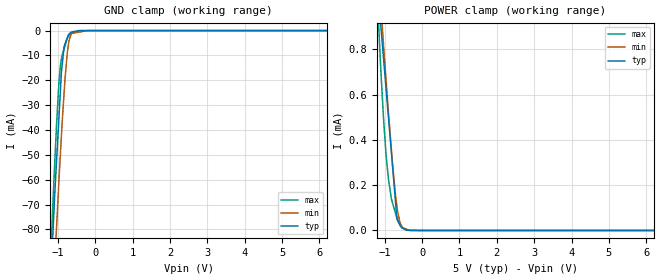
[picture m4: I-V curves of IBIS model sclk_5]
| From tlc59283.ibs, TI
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|   sclk_5 Model
[Model]   sclk_5
Model_type   Input
Vinl = 1.5
Vinh = 3.5
|   typ   min   max
C_comp   5.295e-13   5.058e-13   5.549e-13
| Where nom  PVT is Nominal Process, 5V, 27C
|   Fast PVT is Strong Process,  5.5V, -40C
|   Slow PVT is Weak Process,   4.5V, 125C
[Voltage Range]   5   4.5   5.5
|Ambient Temperature   25   85   -40
|Junction Temperature
[Temperature Range]   27   125   -40
[Power Clamp Reference]   5   4.5   5.5
[GND Clamp Reference]   0   0   0
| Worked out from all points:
|   GND clamp passes 1 mA (typ) near -0.67 V on its own axis
|   POWER clamp passes 1 mA (typ) near -1.15 V on its own axis
[GND Clamp]
|   Voltage   I(typ)   I(min)   I(max)
-5V       -1.598A    -1.521A    -1.69A
-1.373V   -164.7mA   -186.9mA   -158.6mA
-1.14V    -84.95mA   -112.5mA   -73.36mA
-1.122V   -79.17mA   -106.7mA   -66.76mA
-1.034V   -53.01mA   -79.68mA   -38.29mA
-973.5mV  -36.35mA   -61.85mA   -22.17mA
-929.5mV  -24.23mA   -49.72mA   -14.25mA
-900mV    -16.47mA   -41.67mA   -11.16mA
-830mV    -6.402mA   -24.98mA   -7.326mA
-742.5mV  -2.72mA    -8.782mA   -3.153mA
-630mV    -556.8uA   -1.162mA   -1.103mA
10V       0A         0A         0A
[POWER Clamp]
|   Voltage   I(typ)   I(min)   I(max)
-5V       13.71mA    11.48mA    15.23mA
-1.221V   1.234mA    1.281mA    1.114mA
-1.14V    979.4uA    1.086mA    838.7uA
-1.105V   911.1uA    1.003mA    722.3uA
-1.034V   769.5uA    831.2uA    506uA
-968mV    638.8uA    679.5uA    347.5uA
-891mV    486.4uA    506.2uA    218.4uA
-819.5mV  344.8uA    358.9uA    140.6uA
-670mV    48.7uA     104uA      55.32uA
-594mV    26.42uA    38.94uA    24.98uA
-435mV    1.694uA    7.074uA    4.99uA
10V       0A         0A         0A
